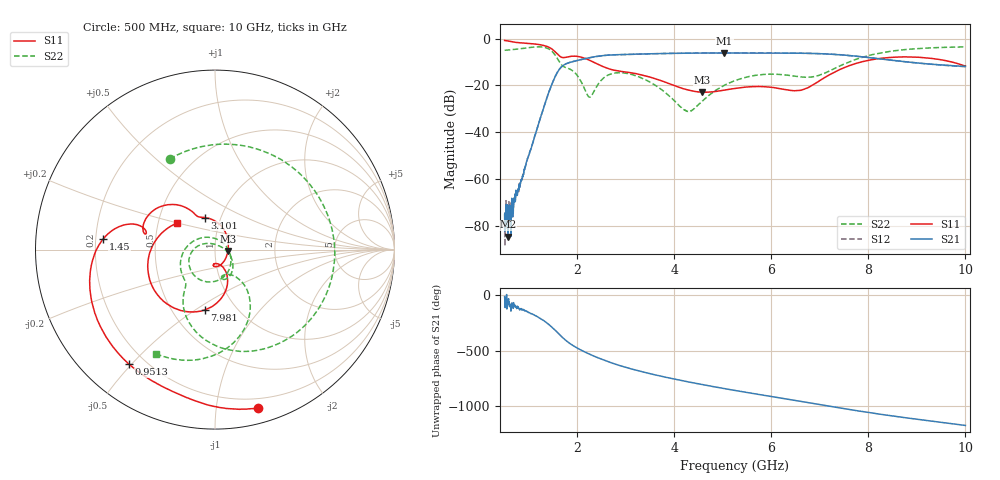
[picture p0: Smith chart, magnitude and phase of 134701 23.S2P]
!  2-Port S-parameters saved by WinCal
! VAR MeasName=S-Parameters (CALIBRATED_DATA) read from VNA (N5242A)
! VAR MeasDate=2013-7-3 16:31:56
! VAR NAME=134701 23
! VAR FILENAME=134701 23.S2P
! VAR DATE=2013-7-3 16:31:56
! VAR PHYS_PORTS=1,2
# Hz S MA R 50
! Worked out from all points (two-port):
!   1601 points, 500 MHz to 10 GHz, reference 50 ohm
!   highest |S21| = -6.13 dB at 5.03 GHz (marker M1); lowest = -84.5 dB at 571.2 MHz (marker M2)
!   |S21| within 3 dB of the highest: 2.035 GHz to 8.446 GHz (6.411 GHz wide, 122 % of centre)
!   lowest |S11| = -22.9 dB at 4.573 GHz (marker M3), VSWR 1.15, Z = 57.7 - j0.916 ohm
!   |S11| at or under -10 dB: 2.332 GHz to 7.847 GHz (5.515 GHz wide, 108 % of centre); 9.723 GHz to end of sweep
!   |S22| runs from -31.2 to -3.5 dB; largest |S21 - S12| = 0.0033
!   S11 on the Smith chart (normalised r, x): 500 MHz: 0.12, -1.30; 951.2 MHz: 0.14, -0.49; 1.45 GHz: 0.23, +0.05; 3.101 GHz: 0.84, +0.31; 7.981 GHz: 0.72, -0.55; 10 GHz: 0.62, +0.20
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5e8  0.9145 -74.8  0.0001763 -11.5  0.000113 -57.7  0.5646 116.6
5.7125e8  0.8913 -84.4  5.959e-05 -59.8  0.0001418 -69.6  0.5718 106.4
9.5125e8  0.7982 -126.9  0.002355 -144.0  0.002264 -147.6  0.6337 42.5
1.206562e9  0.749 -155.5  0.01595 159.6  0.01605 159.7  0.6693 -14.2
1.45e9  0.6247 174.4  0.09162 82.8  0.09151 82.6  0.5659 -81.4
1.71125e9  0.3937 166.5  0.2694 -27.7  0.2687 -27.7  0.2551 -129.6
1.883438e9  0.4217 161.9  0.3191 -86.1  0.3187 -86.1  0.2127 -155.0
2.085312e9  0.4007 145.5  0.3599 -136.5  0.3594 -136.5  0.1168 151.0
2.2575e9  0.3432 132.9  0.3934 -172.6  0.3931 -172.6  0.05643 53.9
2.619688e9  0.2324 120.0  0.4436 123.2  0.4437 123.2  0.1648 -76.9
3.100625e9  0.1869 107.5  0.4644 56.9  0.4638 56.9  0.174 -143.4
3.670625e9  0.1329 73.2  0.4796 -4.9  0.4787 -4.9  0.09129 164.8
4.2525e9  0.08195 25.7  0.4893 -58.7  0.4892 -58.7  0.02843 82.2
4.573125e9  0.0716 -6.3  0.4916 -85.8  0.4919 -85.8  0.04587 10.3
5.030312e9  0.07958 -46.6  0.4936 -122.2  0.494 -122.1  0.1009 -26.6
5.25e9  0.08646 -61.7  0.4927 -138.9  0.4933 -139.0  0.1272 -38.6
6.004062e9  0.09148 -94.8  0.4912 166.0  0.4913 165.9  0.1745 -70.7
6.835312e9  0.09984 -67.4  0.4838 105.7  0.4842 105.8  0.1519 -65.6
7.98125e9  0.3409 -99.6  0.3977 23.4  0.3982 23.2  0.4293 -64.3
8.420625e9  0.3947 -122.9  0.352 -4.8  0.3516 -5.1  0.5297 -78.9
9.222188e9  0.3864 -165.8  0.2891 -51.3  0.2885 -51.6  0.6305 -102.3
1e10  0.2588 145.6  0.2541 -95.0  0.2522 -95.4  0.6655 -119.4
